| TEXAS INSTRUMENTS INCORPORATED
| High Performance Analog Group
| IBIS Model for ads58h40 and ads4449 series of A/D converters
| This file provides unique models under the [Model Selector] for each
| load condition.
| For operation at a specific load condition, select the appropriate model
|after each [Model Selector] keyword.
[IBIS ver]   4.1
[File name]   ads58h40.ibs
[File Rev]   1.2
[Date]   November 08, 2016
[Source]   Model built from TI Spice simulations at:
   Texas Instruments Incorporated.
   Analog-eLab, HPA
   12500 TI Blvd
   Dallas, TX -75243
   For Support e-mail: elab_ibis@list.ti.com
[Notes]   This file contains IBIS Model of various buffers of
   ads58h40 series of A/D converters generated with
   r_fixture of 50 ohm ( 100 ohm differential)
   CLKIN_BUF POWER CLAMP never becomes zero.
   Rev 1.1: 4/23/2013 Added ADS4449 component
   Rev 1.2: 11/08/2016 Correct pin assignments M3,M4,M9,M10
[Disclaimer] This model is designed as an aid for customers of Texas Instruments
   TI and its licensors and suppliers make no warranties, either expressed
   or implied, with respect to this  model, including the warranties of
   merchantability or fitness for a particular purpose.
   The model is provided solely on an "as is" basis. The entire risk as to
   its quality and performance is with the customer.
[Copyright]   (C)Copyright 2016 Texas Instruments Incorporated.
   All rights reserved.
|   Component ads58h40
[Component] ads58h40
[Manufacturer] Texas Instruments.
[Package]
| variable   typ   min   max
R_pkg   0.1600   0.1440   0.1760
L_pkg   5.0000nH   4.5000nH   5.5000nH
C_pkg   2.0000pF   1.8000pF   2.2000pF
[Pin] signal_name   model_name   R_pin   L_pin   C_pin
|   (ohms)   (nH)   (pF)
|	A1	AVDD	power
|	A2	AVDD	power
|	A3	CINM	dummy
|	A4	CINP	dummy
|	A5	AVDD	power
|	A6	VCM	dummy
|	A7	VCM	dummy
|	A8	AVDD	power
|	A9	BINM	dummy
|	A10	BINP	dummy
|	A11	AVDD	power
|	A12	AVDD	power
|	B1	DINP	dummy
|	B2	AVSS	dummy
|	B3	AVDD	power
|	B4	AVDD	power
|	B5	AVSS	dummy
|	B6	AVDD33	power
|	B7	AVDD33	power
|	B8	AVSS	dummy
|	B9	AVDD	power
|	B10	AVDD	power
|	B11	AVSS	dummy
|	B12	AINM	dummy
|	C1	DINM	dummy
|	C2	AVSS	dummy
|	C3	AVSS	dummy
|	C4	AVSS	dummy
|	C5	AVSS	dummy
	C6	CLKINM	clkin
	C7	CLKINP	clkin
|	C8	AVSS	dummy
|	C9	AVSS	dummy
|	C10	AVSS	dummy
|	C11	AVSS	dummy
|	C12	AINP	dummy
|	D1	AVDD	power
|	D2	AVDD	power
|	D3	VCM	dummy
|	D4	AVSS	dummy
|	D5	AVSS	dummy
|	D6	AVSS	dummy
|	D7	AVSS	dummy
|	D8	AVSS	dummy
|	D9	AVSS	dummy
|	D10	VCM	dummy
|	D11	AVDD	power
|	D12	AVDD	power
|	E1	AVDD33	power
|	E2	AVDD33	power
|	E3	NC	dummy
|	E4	DRVSS	dummy
|	E5	DRVSS	dummy
|	E6	DRVSS	dummy
|	E7	DRVSS	dummy
|	E8	DRVSS	dummy
|	E9	DRVSS	dummy
|	E10	PDN	dummy
|	E11	AVDD33	power
|	E12	AVDD33	power
F1	CD13M	dataoutput
F2	CD13P	dataoutput
|	F3	DRVDD	power
|	F4	DRVSS	dummy
|	F5	DRVSS	dummy
|	F6	DRVSS	dummy
|	F7	DRVSS	dummy
|	F8	DRVSS	dummy
|	F9	DRVSS	dummy
|	F10	DRVDD	power
F11	AB13P	dataoutput
F12	AB13M	dataoutput
G1	CD12M	dataoutput
G2	CD12P	dataoutput
|	G3	NC	dummy
|	G4	NC	dummy
|	G5	NC	dummy
|	G6	RESET	dummy
|	G7	SCLK	dummy
|	G8	SDATA	dummy
|	G9	SEN	dummy
G10	SDOUT	cmos_obuf_data
G11	AB12P	dataoutput
G12	AB12M	dataoutput
H1	CD11M	dataoutput
H2	CD11P	dataoutput
H3	CD6P	dataoutput
H4	CD6M	dataoutput
|	H5	DRVDD	power
|	H6	DRVDD	power
|	H7	DRVDD	power
|	H8	DRVDD	power
H9	AB6M	dataoutput
H10	AB6P	dataoutput
H11	AB11P	dataoutput
H12	AB11M	dataoutput
J1	CD10M	dataoutput
J2	CD10P	dataoutput
J3	CD5P	dataoutput
J4	CD5M	dataoutput
J5	CD2P	dataoutput
|	J6	DRVDD	power
|	J7	DRVDD	power
J8	AB2M	dataoutput
J9	AB5M	dataoutput
J10	AB5P	dataoutput
J11	AB10P	dataoutput
J12	AB10M	dataoutput
K1	CD9M	dataoutput
K2	CD9P	dataoutput
K3	CD4P	dataoutput
K4	CD4M	dataoutput
K5	CD2M	dataoutput
|	K6	DRVDD	power
|	K7	DRVDD	power
K8	AB2P	dataoutput
K9	AB4M	dataoutput
K10	AB4P	dataoutput
K11	AB9P	dataoutput
K12	AB9M	dataoutput
L1	CD8M	dataoutput
L2	CD8P	dataoutput
L3	CD3P	dataoutput
L4	CD3M	dataoutput
L5	CD1P	dataoutput
L6	CD1M	dataoutput
L7	AB1M	dataoutput
L8	AB1P	dataoutput
L9	AB3M	dataoutput
L10	AB3P	dataoutput
L11	AB8P	dataoutput
L12	AB8M	dataoutput
M1	CD7M	dataoutput
M2	CD7P	dataoutput
M3	CLKP_CD	clockoutp
M4	CLKM_CD	clockoutm
M5	CD0P	dataoutput
M6	CD0M	dataoutput
M7	AB0M	dataoutput
M8	AB0P	dataoutput
M9	CLKM_AB	clockoutm
M10	CLKP_AB	clockoutp
M11	AB7P	dataoutput
M12	AB7M	dataoutput
[Diff Pin]   inv_pin   vdiff   tdelay_typ   tdelay_min   tdelay_max
C7	C6	350mV	0	0	0
F2	F1	350mV	0	0	0
F11	F12	350mV	0	0	0
G2	G1	350mV	0	0	0
G11	G12	350mV	0	0	0
H2	H1	350mV	0	0	0
H3	H4	350mV	0	0	0
H10	H9	350mV	0	0	0
H11	H12	350mV	0	0	0
J2	J1	350mV	0	0	0
J3	J4	350mV	0	0	0
J5	K5	350mV	0	0	0
J10	J9	350mV	0	0	0
J11	J12	350mV	0	0	0
K2	K1	350mV	0	0	0
K3	K4	350mV	0	0	0
K8	J8	350mV	0	0	0
K10	K9	350mV	0	0	0
K11	K12	350mV	0	0	0
L2	L1	350mV	0	0	0
L3	L4	350mV	0	0	0
L5	L6	350mV	0	0	0
L8	L7	350mV	0	0	0
L10	L9	350mV	0	0	0
L11	L12	350mV	0	0	0
M2	M1	350mV	0	0	0
M3	M4	350mV	0	0	0
M5	M6	350mV	0	0	0
M8	M7	350mV	0	0	0
M10	M9	350mV	0	0	0
M11	M12	350mV	0	0	0
[Series Pin Mapping]  pin_2   model_name
   C6   C7   series_cap
|   Component ads4449
[Component] ads4449
[Manufacturer] Texas Instruments.
[Package]
| variable   typ   min   max
R_pkg   0.1600   0.1440   0.1760
L_pkg   5.0000nH   4.5000nH   5.5000nH
C_pkg   2.0000pF   1.8000pF   2.2000pF
[Pin] signal_name   model_name   R_pin   L_pin   C_pin
	C6	CLKINM	clkin
	C7	CLKINP	clkin
F1	CD13M	dataoutput
F2	CD13P	dataoutput
F11	AB13P	dataoutput
F12	AB13M	dataoutput
G1	CD12M	dataoutput
G2	CD12P	dataoutput
G10	SDOUT	cmos_obuf_data
G11	AB12P	dataoutput
G12	AB12M	dataoutput
H1	CD11M	dataoutput
H2	CD11P	dataoutput
H3	CD6P	dataoutput
H4	CD6M	dataoutput
H9	AB6M	dataoutput
H10	AB6P	dataoutput
H11	AB11P	dataoutput
H12	AB11M	dataoutput
J1	CD10M	dataoutput
J2	CD10P	dataoutput
J3	CD5P	dataoutput
J4	CD5M	dataoutput
J5	CD2P	dataoutput
|	J6	DRVDD	power
|	J7	DRVDD	power
J8	AB2M	dataoutput
J9	AB5M	dataoutput
J10	AB5P	dataoutput
J11	AB10P	dataoutput
J12	AB10M	dataoutput
K1	CD9M	dataoutput
K2	CD9P	dataoutput
K3	CD4P	dataoutput
K4	CD4M	dataoutput
K5	CD2M	dataoutput
|	K6	DRVDD	power
|	K7	DRVDD	power
K8	AB2P	dataoutput
K9	AB4M	dataoutput
K10	AB4P	dataoutput
K11	AB9P	dataoutput
K12	AB9M	dataoutput
L1	CD8M	dataoutput
L2	CD8P	dataoutput
L3	CD3P	dataoutput
L4	CD3M	dataoutput
L5	CD1P	dataoutput
L6	CD1M	dataoutput
L7	AB1M	dataoutput
L8	AB1P	dataoutput
L9	AB3M	dataoutput
L10	AB3P	dataoutput
L11	AB8P	dataoutput
L12	AB8M	dataoutput
M1	CD7M	dataoutput
M2	CD7P	dataoutput
M3	CLKP_AB	clockoutp
M4	CLKM_AB	clockoutm
M5	CD0P	dataoutput
M6	CD0M	dataoutput
M7	AB0M	dataoutput
M8	AB0P	dataoutput
M9	CLKM_CD	clockoutm
M10	CLKP_CD	clockoutp
M11	AB7P	dataoutput
M12	AB7M	dataoutput
[Diff Pin]   inv_pin   vdiff   tdelay_typ   tdelay_min   tdelay_max
C7	C6	350mV	0	0	0
F2	F1	350mV	0	0	0
F11	F12	350mV	0	0	0
G2	G1	350mV	0	0	0
G11	G12	350mV	0	0	0
H2	H1	350mV	0	0	0
H3	H4	350mV	0	0	0
H10	H9	350mV	0	0	0
H11	H12	350mV	0	0	0
J2	J1	350mV	0	0	0
J3	J4	350mV	0	0	0
J5	K5	350mV	0	0	0
J10	J9	350mV	0	0	0
J11	J12	350mV	0	0	0
K2	K1	350mV	0	0	0
K3	K4	350mV	0	0	0
K8	J8	350mV	0	0	0
K10	K9	350mV	0	0	0
K11	K12	350mV	0	0	0
L2	L1	350mV	0	0	0
L3	L4	350mV	0	0	0
L5	L6	350mV	0	0	0
L8	L7	350mV	0	0	0
L10	L9	350mV	0	0	0
L11	L12	350mV	0	0	0
M2	M1	350mV	0	0	0
M3	M4	350mV	0	0	0
M5	M6	350mV	0	0	0
M8	M7	350mV	0	0	0
M10	M9	350mV	0	0	0
M11	M12	350mV	0	0	0
[Series Pin Mapping]  pin_2   model_name
   C6   C7   series_cap
[Model Selector] clockoutp
|The clock output can be in lvds mode or cmos mode. In lvds mode the
|clock signal is a differential signal between pins CLKOUTP and CLKOUTM
|and in cmos mode its a single ended signal at pin CLKOUTP only.
|Note that the model for cmos buffer is different for data and clock output
|buffers whereas the model for the lvds buffer is the same
|  Model name   Description
LVDS_BUF   LVDS 3-state buffer.
|LVDS2X   LVDS 3-state buffer with 2X strength.
|cmos_clk_low   CMOS 3-state (low strength) buffer.
|cmos_clk_low1   CMOS 3-state (low1 strength) buffer.
|cmos_clk_high   CMOS 3-state (high strength) buffer.
|cmos_clk_high1   CMOS 3-state (high1 strength) buffer.
[Model Selector] clockoutm
|When the clock is output in the cmos mode, CLOCKOUTM is SCAN or
|register read. In the lvds mode the clock output is a differential
|signal between pins CLKOUTP and CLKOUTM.
|  Model name   Description
LVDS_BUF   LVDS 3-state buffer.
[Model Selector] dataoutput
|Note that the model for cmos buffer is different for data and clock output
|buffers whereas lvds buffer is the same
|  Model name   Description
LVDS_BUF   LVDS 3-state buffer.
|LVDS2X   LVDS 3-state buffer with 2X strength.
|cmos_data_low   CMOS 3-state (low strength) buffer.
|cmos_data_low1   CMOS 3-state (low1 strength) buffer.
|cmos_data_high   CMOS 3-state (high strength) buffer.
|cmos_data_high1   CMOS 3-state (high1 strength) buffer.
[Model Selector] cmos_obuf_data
|Note that the model for cmos buffer is different for data and clock output
|buffers whereas lvds buffer is the same
|  Model name   Description
|cmos_data_low   CMOS 3-state (low strength) buffer.
|cmos_data_low1   CMOS 3-state (low1 strength) buffer.
|cmos_data_high   CMOS 3-state (high strength) buffer.
CMOS_BUF   CMOS 3-state (high1 strength) buffer.
[Model Selector] clkin
|Note that the model for cmos buffer is different for data and clock output
|buffers whereas lvds buffer is the same
|  Model name   Description
CLKIN_BUF   LVDS input buffer.
|   Model series_cap
[Model]   series_cap
Model_type   Series
C_comp   0.20pF   0.18pF   0.220pF
[Temperature Range]   27.00   125.00   -40.00
[Voltage Range]   1.90V   1.80V   2.0V
[C Series]   2.42pF   1.93pF   2.9pF
| End [Model] series_cap
|End [Component]
|End [Component] ads58h40
| Models and submodels in the file (4): LVDS_BUF (3-state), CMOS_BUF (3-state), CLKIN_BUF (Terminator), series_cap (Series)
